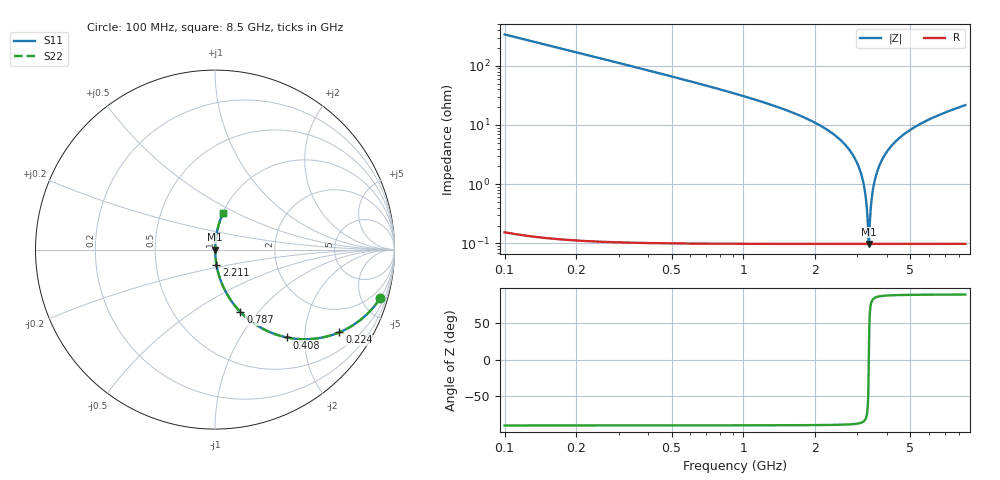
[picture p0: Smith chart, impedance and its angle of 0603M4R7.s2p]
! Created Wed Apr 18 15:53:52 2012
# hz S ma R 50
! 2 Port Network Data from SP1.SP block
! freq  magS11  angS11  magS21  angS21  magS12  angS12  magS22  angS22
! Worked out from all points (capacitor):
!   8401 points, 100 MHz to 8.5 GHz, reference 50 ohm
!   read as one part in series: C = 4.71 pF near 142 MHz
!   lowest |Z| = 98.2 mohm at 3.349 GHz (marker M1)
!   series resonance near 3.349 GHz, so ESL is about 480 pH
!   S11 on the Smith chart (normalised r, x): 100 MHz: 1.00, -6.75; 224 MHz: 1.00, -3.00; 408 MHz: 1.00, -1.63; 787 MHz: 1.00, -0.81; 2.211 GHz: 1.00, -0.17; 8.5 GHz: 1.00, +0.43
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1e8  0.9587 -16.5  0.284 73.5  0.284 73.5  0.9587 -16.5
2.24e8  0.8321 -33.6  0.5541 56.3  0.5541 56.3  0.8321 -33.6
4.08e8  0.6318 -50.7  0.7743 39.2  0.7743 39.2  0.6318 -50.7
7.87e8  0.3756 -67.8  0.9259 22.1  0.9259 22.1  0.3756 -67.8
1.5e9  0.1771 -79.5  0.9832 10.2  0.9832 10.2  0.1771 -79.5
2.211e9  0.08584 -84.4  0.9953 4.9  0.9953 4.9  0.08584 -84.4
2.613e9  0.05051 -86.0  0.9977 2.9  0.9977 2.9  0.05051 -86.0
2.9e9  0.02914 -86.4  0.9986 1.7  0.9986 1.7  0.02914 -86.4
3.069e9  0.01766 -85.8  0.9989 1.0  0.9989 1.0  0.01766 -85.8
3.188e9  0.009999 -83.8  0.999 0.6  0.999 0.6  0.009999 -83.8
3.257e9  0.005716 -79.8  0.999 0.3  0.999 0.3  0.005716 -79.8
3.323e9  0.001864 -58.2  0.999 0.1  0.999 0.1  0.001864 -58.2
3.349e9  0.0009808 -0.8  0.999 0.0  0.999 0.0  0.0009808 -0.8
3.374e9  0.00178 56.5  0.999 -0.1  0.999 -0.1  0.00178 56.5
3.423e9  0.004501 77.2  0.999 -0.3  0.999 -0.3  0.004501 77.2
3.468e9  0.007096 81.7  0.999 -0.4  0.999 -0.4  0.007096 81.7
3.616e9  0.0155 85.5  0.9989 -0.9  0.9989 -0.9  0.0155 85.5
3.886e9  0.03009 86.4  0.9986 -1.7  0.9986 -1.7  0.03009 86.4
4.3e9  0.05086 86.0  0.9977 -2.9  0.9977 -2.9  0.05086 86.0
5.7e9  0.1117 83.1  0.9928 -6.4  0.9928 -6.4  0.1117 83.1
7.1e9  0.164 80.2  0.9855 -9.4  0.9855 -9.4  0.164 80.2
8.5e9  0.2115 77.5  0.9764 -12.2  0.9764 -12.2  0.2115 77.5
